ORGANIZATION_BLOCK "Hardware Interrupt 4"
TITLE =
VERSION : 0.1


VAR_TEMP
  OB44_EV_CLASS : BYTE ;	//Bits 0-3 = 1 (Coming event), Bits 4-7 = 1 (Event class 1)
  OB44_STRT_INF : BYTE ;	//16#41/42/43/44 (Interrupt 1/2/3/4)
  OB44_PRIORITY : BYTE ;	//20 (Priority of 1 is lowest)
  OB44_OB_NUMBR : BYTE ;	//44 (Organization block 44, OB44)
  OB44_RESERVED_1 : BYTE ;	//Reserved for system
  OB44_RESERVED_2 : BYTE ;	//Reserved for system
  OB44_MDL_ADDR : WORD ;	//Base address of module initiating interrupt
  OB44_POINT_ADDR : DWORD ;	//Address of interrupt point on module
  OB44_DATE_TIME : DATE_AND_TIME ;	//Date and time OB44 started
END_VAR
BEGIN
END_ORGANIZATION_BLOCK

